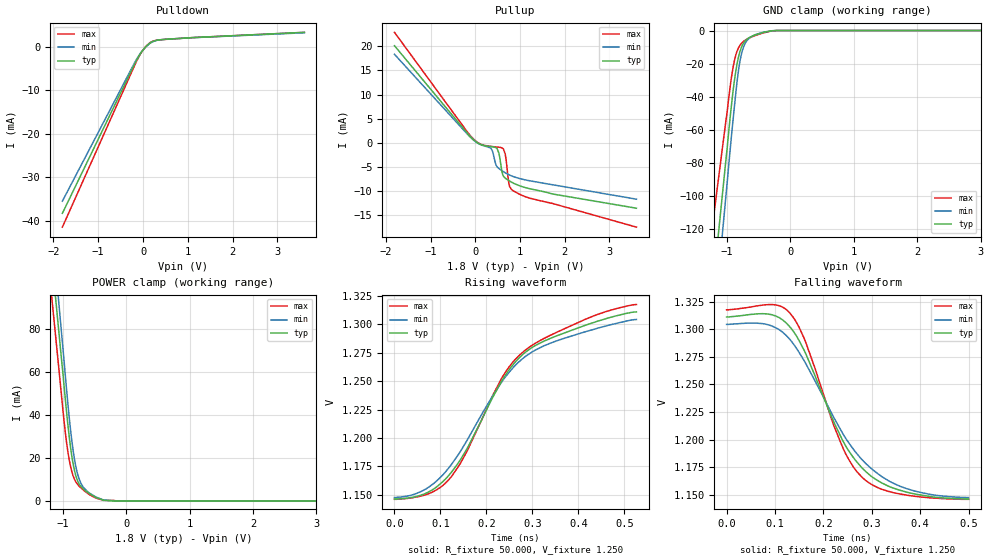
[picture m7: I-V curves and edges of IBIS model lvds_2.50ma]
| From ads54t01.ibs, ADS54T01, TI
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[Model]   lvds_2.50ma
Model_type 3-state
Vref=1.250E+00
Rref=5.000E+01
Cref=0.000E+00
Vmeas=1.250E+00
C_comp   7.860E-13   7.790E-13   7.930E-13
[Voltage Range]   1.800E+00   1.650E+00   1.950E+00
[POWER Clamp Reference]   1.800E+00   1.650E+00   1.950E+00
[GND Clamp Reference]   0.000E+00   0.000E+00   0.000E+00
[Pullup Reference]   1.800E+00   1.650E+00   1.950E+00
[Pulldown Reference]   0.000E+00   0.000E+00   0.000E+00
[Temperature Range]   25   85   -40
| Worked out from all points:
|   slope of the pulldown table from 0 to 0.27 V, typ, clamps not added: 125 ohm
|   slope of the pullup table from 0 to 0.27 V, typ, clamps not added: 263 ohm
|   GND clamp passes 1 mA (typ) near -0.41 V on its own axis
|   POWER clamp passes 1 mA (typ) near -0.41 V on its own axis
|   rising waveform, R_fixture 50.000, V_fixture 1.250: 20-80 % time 153ps typ, 161ps min, 159ps max; typ from 1.15 V to 1.31 V
|   falling waveform, R_fixture 50.000, V_fixture 1.250: 20-80 % time 107ps typ, 128ps min, 87.4ps max; typ from 1.31 V to 1.15 V
[GND Clamp]
-1.8V     -374.4mA   -423.5mA   -288.4mA
-1.02V    -78.69mA   -100.5mA   -54.92mA
-920mV    -41.17mA   -59.34mA   -25.51mA
-860mV    -23.88mA   -36.88mA   -14.48mA
-820mV    -15.94mA   -23.97mA   -10.43mA
-780mV    -10.76mA   -15.27mA   -8.038mA
-740mV    -7.589mA   -9.923mA   -6.562mA
-700mV    -5.657mA   -6.755mA   -5.499mA
-640mV    -4.069mA   -4.329mA   -4.359mA
-460mV    -1.489mA   -1.354mA   -1.806mA
-220mV    -4.201uA   -14.01uA   -11.29uA
3.6V      0A         0A         0A
[Power Clamp]
-1.8V     302.8mA    334.3mA    279.3mA
-1.76V    290.6mA    320.1mA    266.6mA
-1.06V    77.25mA    90.47mA    60.21mA
-940mV    40.5mA     50.88mA    26.54mA
-880mV    24.97mA    33.1mA     16.1mA
-820mV    14.43mA    19.78mA    10.24mA
-780mV    10.23mA    13.83mA    8.195mA
-720mV    6.913mA    8.542mA    6.262mA
-580mV    3.451mA    3.702mA    2.982mA
-360mV    441.4uA    538.8uA    356.5uA
-140mV    0A         9.789uA    18.55uA
3.6V      0A         0A         0A
[Pullup]
-1.81V    20.12mA    18.34mA    22.89mA
-30mV     557.5uA    469.2uA    671.2uA
350mV     -808.5uA   -1.098mA   -745.9uA
490mV     -1.229mA   -4.993mA   -882.3uA
530mV     -2.166mA   -5.344mA   -921.7uA
590mV     -5.599mA   -5.745mA   -1.024mA
630mV     -6.911mA   -5.988mA   -1.288mA
690mV     -7.461mA   -6.32mA    -3.417mA
750mV     -7.826mA   -6.607mA   -8.268mA
810mV     -8.155mA   -6.852mA   -9.67mA
1.73V     -10.61mA   -8.698mA   -12.58mA
3.61V     -13.56mA   -11.69mA   -17.49mA
[Pulldown]
-1.8V     -38.31mA   -35.52mA   -41.49mA
-140mV    -3.033mA   -2.828mA   -3.272mA
-40mV     -1.331mA   -1.265mA   -1.405mA
60mV      -42.79uA   -71.19uA   10uA
160mV     851.3uA    782.6uA    935.5uA
300mV     1.431mA    1.399mA    1.441mA
520mV     1.683mA    1.686mA    1.653mA
3.6V      3.268mA    3.165mA    3.25mA
[Rising Waveform]
R_fixture = 50.000
V_fixture = 1.250
V_fixture_min = 1.250
V_fixture_max = 1.250
|  time   V(typ)   V(min)   V(max)
0s        1.146V     1.147V     1.146V
68ps      1.151V     1.155V     1.15V
120ps     1.168V     1.175V     1.164V
156ps     1.189V     1.197V     1.187V
234ps     1.251V     1.25V      1.253V
260ps     1.266V     1.263V     1.268V
286ps     1.276V     1.272V     1.278V
338ps     1.288V     1.283V     1.29V
428ps     1.301V     1.295V     1.307V
526ps     1.311V     1.304V     1.317V
[Falling Waveform]
R_fixture = 50.000
V_fixture = 1.250
V_fixture_min = 1.250
V_fixture_max = 1.250
|  time   V(typ)   V(min)   V(max)
0s        1.311V     1.304V     1.317V
92ps      1.313V     1.303V     1.322V
134ps     1.3V       1.289V     1.313V
164ps     1.278V     1.269V     1.288V
220ps     1.218V     1.221V     1.215V
242ps     1.198V     1.204V     1.191V
264ps     1.183V     1.19V      1.174V
288ps     1.171V     1.178V     1.163V
372ps     1.152V     1.156V     1.15V
500ps     1.146V     1.147V     1.146V
[Ramp]
dV/dt_r   9.8880E-02/1.5250E-10   9.4080E-02/1.6090E-10   1.0296E-01/1.5850E-10
dV/dt_f   9.8880E-02/1.0691E-10   9.4080E-02/1.2806E-10   1.0296E-01/8.7078E-11
R_load = 50
